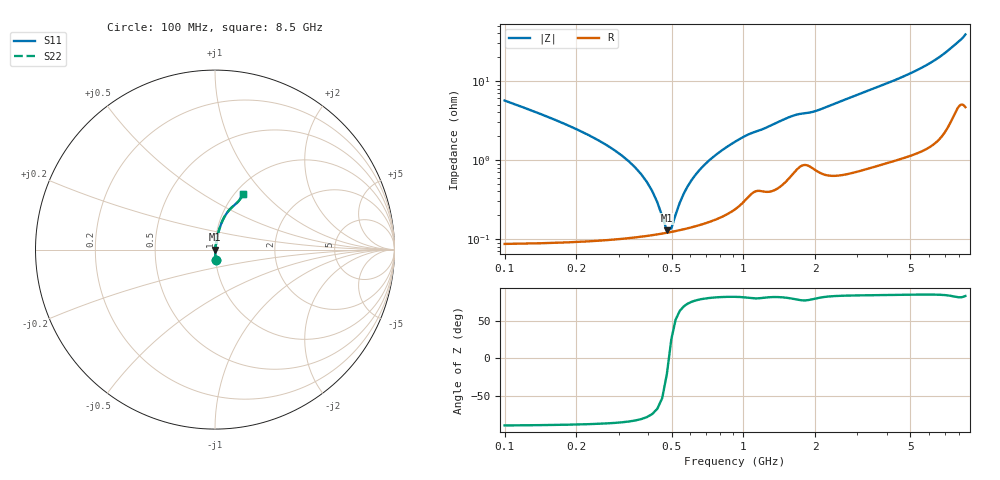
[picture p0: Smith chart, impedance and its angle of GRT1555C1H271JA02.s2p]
!Murata Part Number: GRT1555C1H271JA02
!These Parameters are Measured in Series Mode Connection
!Data Generated on Jun 19, 2026
!  o--ll--o
!Port1  Port2
!  o------o
!Operation Temp=25[degC], DC Bias Voltage=0[V]
!Freq. Start=100[MHz] Stop=9[GHz] 401[Steps]
# Hz S RI R 50
!Freq.(Hz) S11(Real) S11(Imag) S21(Real) S21(Imag) S12(Real) S12(Imag) S22(Real) S22(Imag)
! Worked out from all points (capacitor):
!   401 points, 100 MHz to 8.5 GHz, reference 50 ohm
!   read as one part in series: C = 270 pF near 142 MHz
!   lowest |Z| = 128 mohm at 478 MHz (marker M1)
!   series resonance near 487.1 MHz, so ESL is about 400 pH
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1e8  0.00404 -0.0562  0.996 0.0562  0.996 0.0562  0.00404 -0.0562
1.42e8  0.00232 -0.0379  0.9977 0.0379  0.9977 0.0379  0.00232 -0.0379
3.1e8  0.00113 -0.0113  0.9989 0.0113  0.9989 0.0113  0.00113 -0.0113
3.52e8  0.00111 -0.00798  0.9989 0.00798  0.9989 0.00798  0.00111 -0.00798
3.94e8  0.00112 -0.00516  0.9989 0.00516  0.9989 0.00516  0.00112 -0.00516
4.57e8  0.00117 -0.00154  0.9988 0.00154  0.9988 0.00154  0.00117 -0.00154
4.78e8  0.0012 -0.000452  0.9988 0.000452  0.9988 0.000452  0.0012 -0.000452
4.99e8  0.00123 0.000588  0.9988 -0.000588  0.9988 -0.000588  0.00123 0.000588
5.2e8  0.00126 0.00159  0.9987 -0.00159  0.9987 -0.00159  0.00126 0.00159
5.83e8  0.00138 0.00438  0.9986 -0.00438  0.9986 -0.00438  0.00138 0.00438
6.25e8  0.00148 0.00611  0.9985 -0.00611  0.9985 -0.00611  0.00148 0.00611
6.88e8  0.00164 0.00856  0.9984 -0.00856  0.9984 -0.00856  0.00164 0.00856
7.93e8  0.002 0.0124  0.998 -0.0124  0.998 -0.0124  0.002 0.0124
9.19e8  0.00263 0.0167  0.9974 -0.0167  0.9974 -0.0167  0.00263 0.0167
1.045e9  0.00378 0.0205  0.9962 -0.0205  0.9962 -0.0205  0.00378 0.0205
1.507e9  0.00638 0.0327  0.9936 -0.0327  0.9936 -0.0327  0.00638 0.0327
1.675e9  0.00886 0.0362  0.9911 -0.0362  0.9911 -0.0362  0.00886 0.0362
2.914e9  0.0109 0.063  0.9891 -0.063  0.9891 -0.063  0.0109 0.063
4.3e9  0.0196 0.0987  0.9804 -0.0987  0.9804 -0.0987  0.0196 0.0987
5.707e9  0.0348 0.1447  0.9652 -0.1447  0.9652 -0.1447  0.0348 0.1447
7.114e9  0.0728 0.2125  0.9272 -0.2125  0.9272 -0.2125  0.0728 0.2125
8.5e9  0.1579 0.309  0.8421 -0.309  0.8421 -0.309  0.1579 0.309
